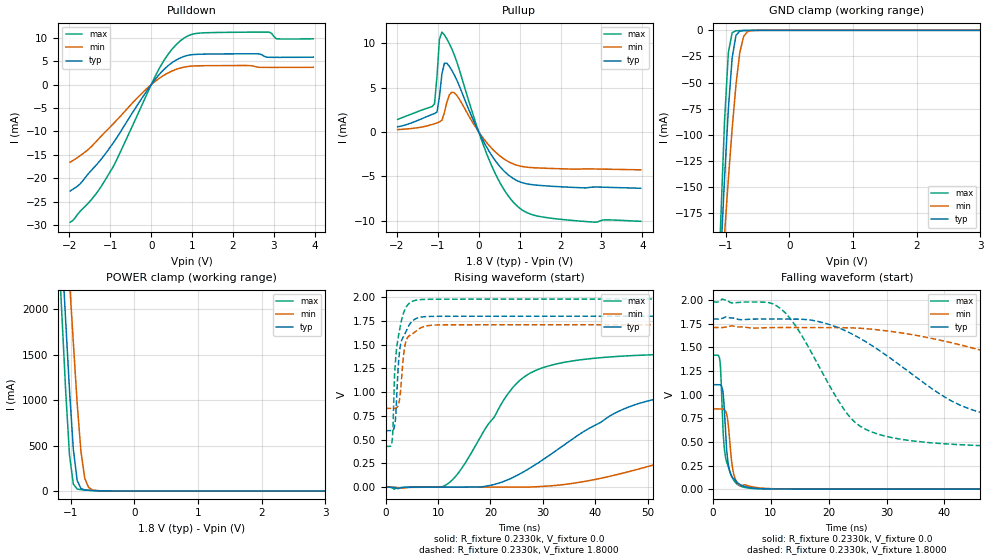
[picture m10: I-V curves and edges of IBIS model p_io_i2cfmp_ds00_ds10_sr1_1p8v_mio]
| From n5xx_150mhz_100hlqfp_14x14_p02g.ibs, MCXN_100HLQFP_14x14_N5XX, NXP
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[Model] p_io_i2cfmp_ds00_ds10_sr1_1p8v_mio
|   Model p_io_i2cfmp_ds00_ds10_sr1_1p8v_mio
| This model was characterised for following simulation conditions:
| External (pad) voltage:
|   - Typ: 1.8V,   - Min: 1.71V,   - Max: 1.98V
| Library cells for typ/min/max conditions are connected as defined below:
|  pad - External Pad
|  ipp_do_lv - Core Input
|  ipp_obe_lv - Output Buffer Enable
|  IOGC - NC
|  REFH3V3 - REFH3V3
|  REFL3V3 - REFL3V3
|  ZI - NC
|  abut_ncal_vddio[1] - vssio vddio vddio
|  abut_ncal_vddio[2] - vddio vddio vssio
|  abut_ncal_vddio[3] - vddio
|  abut_ncal_vddio[4] - vssio vddio vddio
|  abut_ncal_vddio[5] - vddio vddio vssio
|  abut_ncal_vddio[6] - vddio
|  abut_pcal_vddio[1] - vssio
|  abut_pcal_vddio[2] - vddio vssio vddio
|  abut_pcal_vddio[3] - vssio
|  abut_pcal_vddio[4] - vssio
|  abut_pcal_vddio[5] - vddio vssio vddio
|  abut_pcal_vddio[6] - vssio
|  ipp_do_1p8v - ipp_do_1p8v
|  ipp_dse_lv[0] - 0
|  ipp_dse_lv[1] - 0
|  ipp_eftd_lv - NC
|  ipp_ina_mux_vddio - NC
|  ipp_ina_mux_vddio[0] - NC
|  ipp_ina_mux_vddio[1] - NC
|  ipp_ina_r0_vddio - NC
|  ipp_ina_r0a_vddio - NC
|  ipp_ina_r0b_vddio - NC
|  ipp_ina_r0c_vddio - NC
|  ipp_ina_r0d_vddio - NC
|  ipp_ina_r0e_vddio - NC
|  ipp_ina_r0f_vddio - NC
|  ipp_ina_r300_vddio - NC
|  ipp_ina_r300a_vddio - NC
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Model_type I/O
Polarity   Non-Inverting
Enable   Active-High
Vinl =   0.5400V
Vinh =   1.2600V
Vmeas =  0.9000V
Cref =   30.0000pF
Rref =   1.0000M
Vref =   1.8000V
C_comp   1.7515pF   1.7218pF   1.7928pF
|C_comp_pullup   0.7576pF   0.8231pF   0.7013pF
|C_comp_pulldown   0.8800pF   0.8507pF   0.9093pF
[Model Spec]
| variable   typ   min   max
Vinh   1.2600V   1.1970V   1.3860V
Vinl   0.5400V   0.5130V   0.5940V
[Temperature Range]   25.0000   0.1250k   -40.0000
[Voltage Range]   1.8000V   1.7100V   1.9800V
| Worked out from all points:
|   slope of the pulldown table from 0 to 0.27 V, typ, clamps not added: 94.2 ohm
|   slope of the pullup table from 0 to 0.27 V, typ, clamps not added: 117 ohm
|   GND clamp passes 1 mA (typ) near -0.78 V on its own axis
|   POWER clamp passes 1 mA (typ) near -0.53 V on its own axis
|   rising waveform, R_fixture 0.2330k, V_fixture 0.0: 20-80 % time 20.4ns typ, 38.4ns min, 10.3ns max; typ from 0 V to 1.1 V
|   rising waveform, R_fixture 0.2330k, V_fixture 1.8000: 20-80 % time 1.14ns typ, 1.04ns min, 1.25ns max; typ from 0.594 V to 1.8 V
|   falling waveform, R_fixture 0.2330k, V_fixture 0.0: 20-80 % time 854ps typ, 899ps min, 983ps max; typ from 1.1 V to 0 V
|   falling waveform, R_fixture 0.2330k, V_fixture 1.8000: 20-80 % time 18.6ns typ, 36.3ns min, 9.12ns max; typ from 1.8 V to 0.595 V
[Pulldown]
|Voltage   I(typ)   I(min)   I(max)
-1.98V    -22.71mA   -16.55mA   -29.37mA
-1.74V    -21.21mA   -15.2mA    -27.08mA
-1.14V    -15mA      -10.25mA   -20.59mA
-900mV    -12.1mA    -8.114mA   -17.06mA
180mV     2.012mA    1.246mA    3.179mA
420mV     4.088mA    2.535mA    6.549mA
720mV     5.743mA    3.561mA    9.405mA
1.08V     6.453mA    4.005mA    10.9mA
1.74V     6.558mA    4.067mA    11.15mA
2.88V     5.839mA    3.677mA    11.2mA
3.06V     5.829mA    3.677mA    9.802mA
3.96V     5.871mA    3.703mA    9.79mA
[Pullup]
|Voltage   I(typ)   I(min)   I(max)
-1.98V    578.3uA    262.5uA    1.413mA
-1.08V    2.082mA    925.3uA    3.166mA
-1.02V    2.24mA     1.021mA    6.246mA
-960mV    3.967mA    1.121mA    10.46mA
-900mV    6.538mA    1.314mA    11.26mA
-840mV    7.737mA    2.17mA     10.95mA
-780mV    7.751mA    3.329mA    10.49mA
-600mV    6.46mA     4.424mA    8.721mA
240mV     -2.08mA    -1.452mA   -2.99mA
900mV     -5.408mA   -3.707mA   -8.19mA
1.74V     -6.118mA   -4.117mA   -9.719mA
3.96V     -6.358mA   -4.279mA   -10.08mA
[GND_clamp]
|Voltage   I(typ)   I(min)   I(max)
-1.98V    -1.571A    -1.243A    -2.046A
-1.14V    -296.8mA   -307.7mA   -291.9mA
-1.08V    -217.1mA   -250.6mA   -183.3mA
-1.02V    -142mA     -195.3mA   -87.29mA
-960mV    -75.42mA   -142.6mA   -21.4mA
-900mV    -26.21mA   -93.87mA   -2.23mA
-840mV    -4.776mA   -51.84mA   -446.5uA
-780mV    -725.4uA   -21.22mA   -243.9uA
-720mV    -200uA     -5.88mA    -159.3uA
-660mV    -98.47uA   -1.291mA   -98.82uA
-420mV    -3.926uA   -10.95uA   -2.45uA
3.96V     0A         0A         0A
[POWER_clamp]
|Voltage   I(typ)   I(min)   I(max)
-1.98V    13.51A     13.25A     14.01A
-1.2V     3.414A     4.356A     2.802A
-1.14V    2.644A     3.675A     1.949A
-1.08V    1.876A     2.995A     1.103A
-1.02V    1.113A     2.317A     397.9mA
-960mV    462.1mA    1.641A     75.38mA
-900mV    117mA      972.3mA    21.31mA
-840mV    26.38mA    432.6mA    13.76mA
-780mV    10.65mA    139.4mA    9.996mA
-720mV    6.506mA    38.48mA    6.892mA
-660mV    4.142mA    12.01mA    4.303mA
3.96V     0A         0A         0A
[Ramp]
| variable   typ   min   max
dV/dt_r  0.6630/20.3846n   0.5069/38.3620n   0.8506/10.2935n
dV/dt_f  0.7233/18.5806n   0.5260/36.2767n   0.9306/9.1221n
R_load = 0.2330k
[Rising Waveform]
R_fixture= 0.2330k
V_fixture= 0.0
V_fixture_min= 0.0
V_fixture_max= 0.0
|time   V(typ)   V(min)   V(max)
0s        1.278nV    605.2nV    30.99pV
11.63ns   -71.37uV   -35.28uV   27.79mV
19.17ns   10.47mV    -17.62uV   629.9mV
25.29ns   130mV      377.2uV    1.109V
37.76ns   584.6mV    57.91mV    1.345V
45.64ns   828mV      152.9mV    1.381V
54.11ns   955.7mV    281.7mV    1.399V
72.11ns   1.051V     552.9mV    1.413V
92.13ns   1.085V     715.4mV    1.417V
210.6ns   1.105V     844.8mV    1.418V
[Rising Waveform]
R_fixture= 0.2330k
V_fixture= 1.8000
V_fixture_min= 1.7100
V_fixture_max= 1.9800
|time   V(typ)   V(min)   V(max)
0s        594.4mV    829.2mV    429mV
1.253ns   594.5mV    829.3mV    489.7mV
1.401ns   597.9mV    829.3mV    609.7mV
1.757ns   654.4mV    829.1mV    1.217V
2.493ns   1.325V     875.7mV    1.601V
2.973ns   1.529V     1.085V     1.74V
3.441ns   1.588V     1.391V     1.835V
3.923ns   1.643V     1.54V      1.895V
6.156ns   1.782V     1.658V     1.971V
210.6ns   1.8V       1.71V      1.98V
[Falling Waveform]
R_fixture= 0.2330k
V_fixture= 0.0
V_fixture_min= 0.0
V_fixture_max= 0.0
|time   V(typ)   V(min)   V(max)
0s        1.105V     848.6mV    1.418V
1.191ns   1.105V     847.9mV    1.355V
1.343ns   1.1V       848.1mV    1.22V
1.748ns   1.008V     848.1mV    588.6mV
2.259ns   488.6mV    810.4mV    305.2mV
2.807ns   207.3mV    564.9mV    202.7mV
3.262ns   128.8mV    266.9mV    131.4mV
3.712ns   104.3mV    128mV      81.8mV
6.175ns   18.17mV    33.2mV     10.91mV
210.6ns   372.3nV    4.133uV    90.37nV
[Falling Waveform]
R_fixture= 0.2330k
V_fixture= 1.8000
V_fixture_min= 1.7100
V_fixture_max= 1.9800
|time   V(typ)   V(min)   V(max)
0s        1.8V       1.71V      1.98V
11.38ns   1.8V       1.709V     1.922V
14.41ns   1.798V     1.71V      1.714V
24.39ns   1.629V     1.705V     715.9mV
34.77ns   1.199V     1.63V      508.3mV
42.2ns    902.7mV    1.534V     471.6mV
50.33ns   757mV      1.4V       452.3mV
67.83ns   656.2mV    1.108V     436.2mV
85.86ns   621.3mV    965.6mV    431.3mV
210.6ns   594.6mV    833.3mV    429mV
